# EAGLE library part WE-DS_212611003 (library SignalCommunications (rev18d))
WE-DS D-SUB-Filter, Solder Pin Straight Characteristics Standard type filtered with 1000 pF High attenuation: max. ≥ 40 dB @ 180 MHz Choice of UNC 4/40 or through hole Rated voltage: 100 VDC Rated current @ 20 ºC: 5 A Withstand voltage: 250 VRMS Insulation resistance: min. 1000 MΩ Operating temperature: –55 ºC to +125 ºC Applications Filtering of interfaces External connection to -printer -sensor -display Details see: http://katalog.we-online.de/en/pbs/Filter_gerade Created on 2015-05-04 2015 (C) Wurth Elektronik
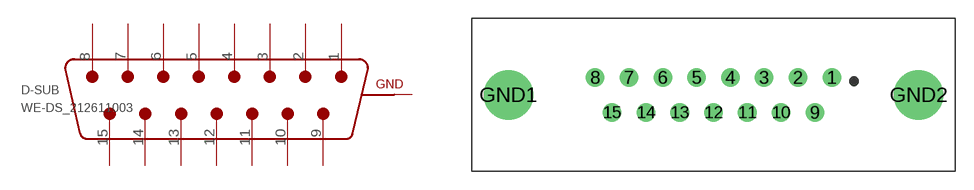
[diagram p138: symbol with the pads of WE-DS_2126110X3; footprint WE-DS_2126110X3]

Designator prefix D-SUB

## WE-DS_212611003 (WE-NUMBER: 212611003/15pins_female)  [WE-DS_2126110X3]
1  8  pas
2  7  pas
3  6  pas
4  5  pas
5  4  pas
6  3  pas
7  2  pas
8  1  pas
9  15  pas
10  14  pas
11  13  pas
12  12  pas
13  11  pas
14  10  pas
15  9  pas
GND1  GND  pas
GND2  GND  pas

## Footprint WE-DS_2126110X3 (pad centres in mm)
drill 1: 1 9.6,1.42; 2 6.86,1.42; 3 4.11,1.42; 4 1.37,1.42; 5 -1.37,1.42; 6 -4.11,1.42; 7 -6.86,1.42; 8 -9.6,1.42; 9 8.23,-1.42; 10 5.48,-1.42; 11 2.74,-1.42; 12 0,-1.42; 13 -2.74,-1.42; 14 -5.48,-1.42; 15 -8.23,-1.42
drill 3: GND1 -16.65,0; GND2 16.65,0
